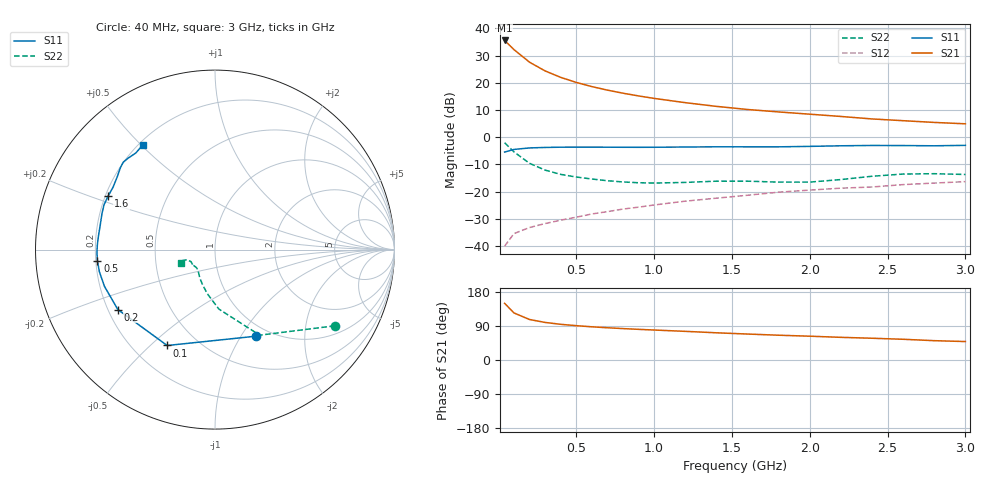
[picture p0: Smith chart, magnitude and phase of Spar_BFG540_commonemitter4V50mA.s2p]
! Filename:  BFG540X.S2P  Version:  3.0
! NXP part #: BFG540  Date: Feb 1992
! Bias condition: Vce=4V, Ic=50mA
! IN LINE PINNING: same data as with cross emitter pinning.
#  MHz  S  MA  R  50
! Freq  S11  S21  S12  S22  !GUM [dB]
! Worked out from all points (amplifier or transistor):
!   21 points, 40 MHz to 3 GHz, reference 50 ohm
!   highest |S21| = 35.5 dB at 40 MHz (marker M1)
!   |S21| within 3 dB of that: start of sweep to 93.7 MHz
!   unconditionally stable (mu >= 1): 619.6 MHz to end of sweep
!   at 300 MHz: K = 0.74, MSG = 28.0 dB, |S12| = -31.7 dB
!   at 1 GHz: K = 1.14, MAG = 17.3 dB, |S12| = -24.9 dB
!   at 3 GHz: K = 1.14, MAG = 8.3 dB, |S12| = -16.3 dB
!   S11 on the Smith chart (normalised r, x): 40 MHz: 0.86, -1.17; 100 MHz: 0.34, -0.57; 200 MHz: 0.24, -0.27; 500 MHz: 0.21, -0.05; 1.6 GHz: 0.21, +0.23; 3 GHz: 0.22, +0.51
40  0.534 -64.6  59.74 149.6  0.01 65.9  0.792 -32.4
100  0.597 -116.5  40.62 124.2  0.017 50.6  0.538 -62.4
200  0.636 -148.3  23.84 106.9  0.022 47.2  0.332 -86.3
300  0.649 -161.6  16.5 99.1  0.026 49.4  0.249 -100.0
400  0.656 -169.2  12.56 94.2  0.03 53.3  0.208 -109.3
500  0.658 -174.6  10.14 90.6  0.034 56.2  0.186 -115.8
600  0.658 -178.8  8.509 87.6  0.039 59.4  0.171 -120.7
700  0.656 177.6  7.325 85.1  0.043 61.4  0.159 -124.9
800  0.654 174.2  6.434 82.9  0.048 62.9  0.151 -128.7
900  0.653 170.9  5.729 80.9  0.052 64.7  0.146 -132.8
1000  0.654 167.7  5.164 79.1  0.057 65.9  0.144 -136.8
1200  0.661 162.3  4.312 75.6  0.067 67.2  0.148 -142.5
1400  0.667 157.9  3.685 71.8  0.076 67.4  0.156 -144.0
1600  0.666 153.5  3.229 68.5  0.086 68.6  0.156 -144.2
1800  0.666 148.5  2.912 65.4  0.098 68.1  0.15 -146.8
2000  0.679 143.3  2.647 62.8  0.107 68.5  0.15 -153.7
2200  0.696 139.4  2.405 59.8  0.116 68.0  0.167 -160.2
2400  0.706 136.5  2.166 57.4  0.122 68.4  0.192 -161.4
2600  0.703 133.7  2.011 54.7  0.135 67.1  0.211 -158.7
2800  0.696 129.3  1.869 51.0  0.144 64.6  0.214 -156.1
3000  0.709 124.4  1.763 48.7  0.153 64.9  0.207 -158.1
